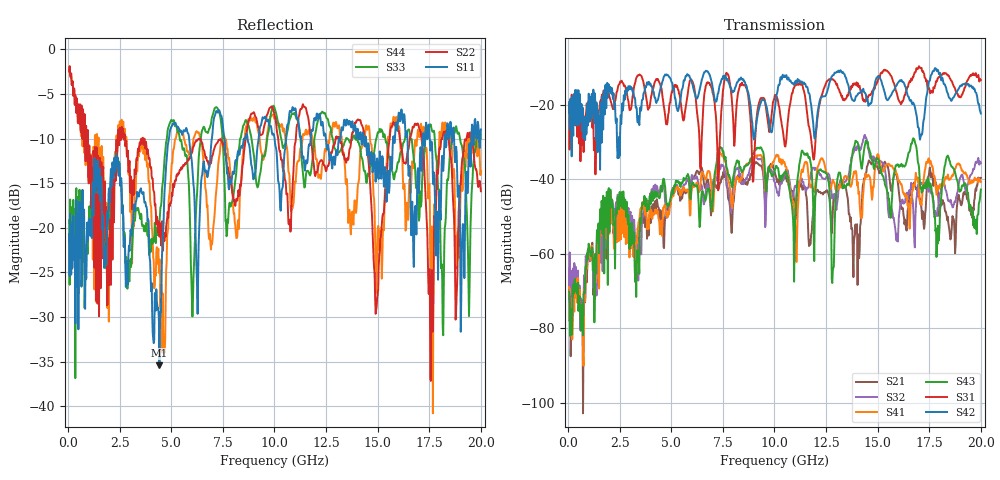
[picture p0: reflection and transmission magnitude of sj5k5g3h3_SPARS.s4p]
! FILE: E:\users\goganessyan\GBX_Backplane\FR408_backplane\1m_INBOUND_NEXT\sj5k5g3h3_SPARS.s4p
# MHZ S RI R 50.00
! FREQ  S11  S12  S13  S14
!  S21  S22  S23  S24
!  S31  S32  S33  S34
!  S41  S42  S43  S44
!  REAL  IMAG  REAL  IMAG  REAL  IMAG  REAL  IMAG
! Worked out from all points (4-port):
!   799 points, 50 MHz to 20 GHz, reference 50 ohm
!   strongest paths, dB at 50 MHz, 5.025 GHz, 10.03 GHz, 15.03 GHz, 20 GHz:
!     S42: -19.3, -14.1, -20.5, -12.4, -22.4
!     S31: -19.7, -16.6, -17.4, -13.3, -13.4
!     S43: -70.3, -44.2, -37.4, -34.7, -42.8
!     S41: -69.0, -45.0, -34.3, -33.3, -40.7
!     S32: -68.8, -43.6, -41.0, -35.9, -35.7
!     S21: -64.2, -43.0, -38.4, -37.4, -39.7
!   lowest |S11| = -35.4 dB at 4.425 GHz (marker M1), VSWR 1.03, Z = 51 + j1.4 ohm
!   |S11| at or under -10 dB: start of sweep to 4.887 GHz; 5.863 GHz to 6.966 GHz (1.104 GHz wide, 17.2 % of centre); 14.43 GHz to 15.75 GHz (1.313 GHz wide, 8.7 % of centre)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
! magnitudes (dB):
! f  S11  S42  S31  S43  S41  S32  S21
! 50 MHz  -20.7  -19.3  -19.7  -70.3  -69.0  -68.8  -64.2
! 4.425 GHz  -35.4  -16.9  -14.0  -45.1  -52.1  -44.1  -50.7
! 8.975 GHz  -14.6  -28.6  -40.5  -33.3  -34.8  -34.6  -36.8
! 12.5 GHz  -10.3  -17.3  -14.3  -38.4  -38.0  -39.7  -43.4
! 12.82 GHz  -12.7  -12.1  -13.2  -64.5  -40.2  -44.9  -48.4
! 13.97 GHz  -10.0  -17.7  -14.0  -30.0  -39.0  -31.2  -53.2
! 20 GHz  -9.0  -22.4  -13.4  -42.8  -40.7  -35.7  -39.7
